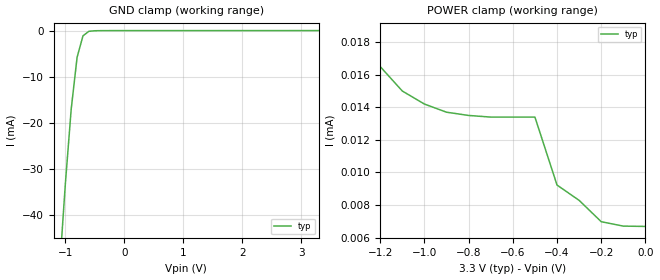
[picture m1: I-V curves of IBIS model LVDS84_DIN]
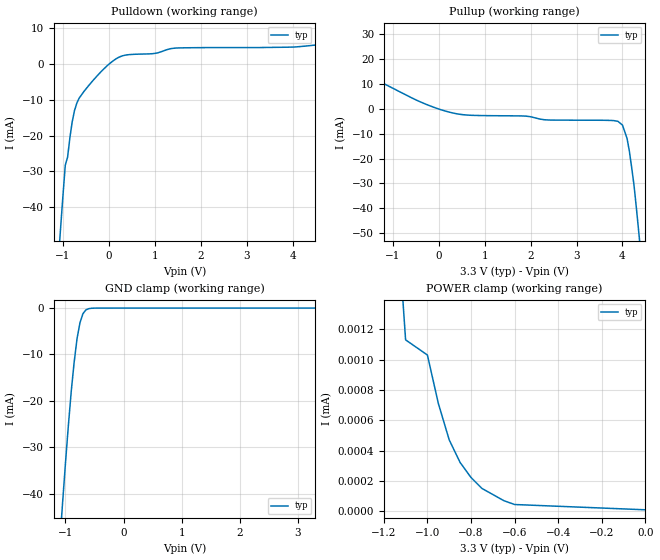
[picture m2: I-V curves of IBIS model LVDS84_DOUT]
|   Texas Instruments Incorporated
|   Data Transmissions Products
|   IBIS Model for SN75LVDS84
|   48DGG Package
[IBIS Ver]   2.1
[Comment char]   |_char
[File name]   75lvds84.ibs
[File Rev]   2.0
[Date]   21Feb97
[Source]   File originated at Texas Instruments Incorporated.
   Data Transmission Products Group. All data based on
   Empirical Measurements(Bench).
[Notes]   File created by Thomas Fisher
[Disclaimer]
(C) Copyright Texas Instruments Incorporated 1997
   All rights reserved
  Texas Instruments Incorporated hereby grants the user of this IBIS
model a non-exclusive, nontransferable license to use this IBIS model
under the following terms.  Before using this IBIS model, the user
should read this license.  If the user does not accept these terms,
the IBIS model should be returned to Texas Instruments within 30 days.
  The user is granted this license only to use the IBIS model and
is not granted rights to sell, load, rent, lease or license the IBIS
model in whole or in part, or in modified form to anyone other than
user.  User may modify the IBIS model to suit its specific applications
but rights to derivative works and such modifications shall belong to
Texas Instruments.
  This IBIS model is provided on an "AS IS" basis and Texas Instruments
makes absolutely no warranty with respect to the information contained
herein.  TEXAS INSTRUMENTS DISCLAIMS AND CUSTOMER WAIVES ALL WARRANTIES,
EXPRESS OR IMPLIED, INCLUDING WARRANTIES OF MERCHANTABILITY OR FITNESS
FOR A PARTICULAR PURPOSE. The entire risk as to quality and performance
is with the Customer. ACCORDINGLY, IN NO EVENT SHALL THE COMPANY BE LIABLE
FOR ANY DAMAGES, WHETHER IN CONTRACT OR TORT,INCLUDING ANY LOST PROFITS
OR OTHER INCIDENTAL, CONSEQUENTIAL, EXEMPLARY, OR PUNITIVE DAMAGES ARISING
OUT OF THE USE OR APPLICATION OF THE IBIS model provided in this package.
Further, Texas Instruments reserves the right to discontinue or make changes
without notice to any product herein to improve reliability, function, or
design. Texas Instruments does not convey any license under patent rights
or any other intellectual property rights, including those of third parties.
Contact Texas Instruments at ATTN:DATA TRANSMISSIONS
Thomas Fisher  8505 Forest Lane, M/S 8710, Dallas, TX 75243-4136
IBIS Open Forum disclaims all warranties. See DISCLAIM.TXT
in vhdl.org:/pub/IBIS/models for the full disclaimer.
[Copyright]   Copyright 1997, Texas Instruments, All Rights Reserved
[Component]   SN75LVDS84DGG
[Manufacturer]  Texas Instruments Incorporated
[Package]
|   typ   min   max
R_pkg   0.036   0.022   0.041
L_pkg   2.128nH   2.045nH   2.336nH
C_pkg   0.357pF   0.310pF   0.394pF
[Pin]  signal_name   model_name   R_pin   L_pin   C_pin
1   D4   LVDS84_DIN   0.041   2.221n   0.310p
2   VCC   POWER   0.041   2.297n   0.394p
3   D5   LVDS84_DIN   0.022   2.336n   0.380p
4   D6   LVDS84_DIN   0.031   2.056n   0.343p
5   GND   GND   0.034   2.099n   0.383p
6   D7   LVDS84_DIN   0.034   2.046n   0.360p
7   D8   LVDS84_DIN   0.036   2.052n   0.354p
8   VCC   POWER   0.038   2.081n   0.354p
9   D9   LVDS84_DIN   0.039   2.091n   0.353p
10   D10   LVDS84_DIN   0.039   2.068n   0.349p
11   GND   GND   0.039   2.098n   0.361p
12   D11   LVDS84_DIN   0.039   2.100n   0.343p
13   D12   LVDS84_DIN   0.039   2.100n   0.343p
14   VCC   POWER   0.039   2.098n   0.361p
15   D13   LVDS84_DIN   0.039   2.068n   0.349p
16   D14   LVDS84_DIN   0.039   2.091n   0.353p
17   GND   GND   0.038   2.081n   0.354p
18   D15   LVDS84_DIN   0.036   2.052n   0.354p
19   D16   LVDS84_DIN   0.034   2.045n   0.360p
20   D17   LVDS84_DIN   0.034   2.099n   0.383p
21   VCC   POWER   0.031   2.056n   0.343p
22   D18   LVDS84_DIN   0.022   2.330n   0.381p
23   D19   LVDS84_DIN   0.041   2.294n   0.394p
24   GND   GND   0.041   2.220n   0.310p
25   D20   LVDS84_DIN   0.041   2.221n   0.310p
26   CLKIN   LVDS84_DIN   0.041   2.295n   0.394p
27   SHTDN   LVDS84_DIN   0.022   2.333n   0.378p
28   PLLGND   GND   0.031   2.056n   0.343p
29   PLLVCC   POWER   0.034   2.097n   0.385p
30   PLLGND   GND   0.034   2.045n   0.360p
31   LVDSGND   GND   0.036   2.052n   0.354p
32   CLKOUTP   LVDS84_DOUT   0.038   2.080n   0.354p
33   CLKOUTM   LVDS84_DOUT   0.039   2.090n   0.352p
34   Y2P   LVDS84_DOUT   0.039   2.067n   0.349p
35   Y2M   LVDS84_DOUT   0.039   2.097n   0.362p
36   LVDSGND   GND   0.039   2.100n   0.343p
37   LVDSVCC   POWER   0.039   2.100n   0.343p
38   Y1P   LVDS84_DOUT   0.039   2.097n   0.362p
39   Y1M   LVDS84_DOUT   0.039   2.067n   0.349p
40   Y0P   LVDS84_DOUT   0.039   2.090n   0.352p
41   Y0M   LVDS84_DOUT   0.038   2.080n   0.354p
42   LVDSGND   GND   0.036   2.052n   0.354p
43   NC   NC
44   D0   LVDS84_DIN   0.034   2.097n   0.385p
45   D1   LVDS84_DIN   0.031   2.056n   0.343p
46   GND   GND   0.022   2.335n   0.377p
47   D2   LVDS84_DIN   0.041   2.297n   0.394p
48   D3   LVDS84_DIN   0.041   2.221n   0.310p
[Diff_pin]   inv_pin   vdiff   tdelay_typ   tdelay_min   tdelay_max
| The 'YXP' pin is Diff_pin and the 'YXM' pin is the inv_pin
| The 'CLKOUTP' pin is Diff_pin and the 'CLKOUTM' pin is the inv_pin
32   33   NA   0 0 0
34   35   NA   0 0 0
38   39   NA   0 0 0
40   41   NA   0 0 0
| Models and submodels in the file (2): LVDS84_DIN (Input), LVDS84_DOUT (3-state)
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|   Driver Input  MODEL
[Model]   LVDS84_DIN
Model_type   Input
|Signals   D0,D1,D2,D3,D4,D5,D6,D7,D8,D9,D10,D11,D12,D13,D14,D15,D16,
|   D17,D18,D19,D20,SHTDN,CLKIN
Vinh = 2.0
Vinl = 0.8
|   typ   min   max
C_comp   1.0pF   NA   NA
|   typ   min   max
[Temperature Range]   25.0   NA   NA
[Voltage range]   3.3V   3.0V   3.6V
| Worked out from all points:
|   GND clamp passes 1 mA (typ) near -0.69 V on its own axis
[Power_clamp]
| Note that the[POWER_clamp]voltage table is referenced to Vcc
| and is calculated using Vtable=Vcc - Vmeasured.
|   Voltage   I(typ)   I(min)   I(max)
-3.3V     780uA      NA         NA
-1.3V     19.1uA     NA         NA
-1.2V     16.5uA     NA         NA
-1.1V     15uA       NA         NA
-1V       14.2uA     NA         NA
-900mV    13.7uA     NA         NA
-800mV    13.5uA     NA         NA
-500mV    13.4uA     NA         NA
-400mV    9.23uA     NA         NA
-300mV    8.29uA     NA         NA
-200mV    6.98uA     NA         NA
0V        6.69uA     NA         NA
[GND_clamp]
|   Voltage   I(typ)   I(min)   I(max)
-3.3V     -485.8mA   NA         NA
-1.1V     -52.3mA    NA         NA
-1V       -33.38mA   NA         NA
-900mV    -17.03mA   NA         NA
-800mV    -5.78mA    NA         NA
-700mV    -1.13mA    NA         NA
-600mV    -150uA     NA         NA
-300mV    -2.96uA    NA         NA
3.3V      6.69uA     NA         NA
|   Driver Output  MODEL
[Model]   LVDS84_DOUT
Model_type   3-state
| Signals   Y0P,Y0M,Y1P,Y1M,Y2P,Y2M,CLKOUTP,CLKOUTM
Vmeas = 1.2V   |Reference voltage for timing measurements
Cref = 5pF   |Timing specification test load capacitance value
Rref = 50   |Note: 50 Ohm load; single ended configuration
Vref = 1.18V   |Timing specification test load voltage
| variable   typ   min   max
C_comp   1.0pF   NA   NA
|   typ   min   max
[Temperature Range]   25.0   NA   NA
[Voltage range]   3.3V   3.0V   3.6V
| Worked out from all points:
|   slope of the pulldown table from 0 to 0.495 V, typ, clamps not added: 182 ohm
|   slope of the pullup table from 0 to 0.495 V, typ, clamps not added: 224 ohm
|   GND clamp passes 1 mA (typ) near -0.69 V on its own axis
[Pulldown]
|   Voltage   I(typ)   I(min)   I(max)
-3.3V     -466.3mA   NA         NA
-1.1V     -54.41mA   NA         NA
-1.05V    -45.42mA   NA         NA
-950mV    -28.23mA   NA         NA
-900mV    -26.02mA   NA         NA
-800mV    -16.18mA   NA         NA
-700mV    -10.96mA   NA         NA
-250mV    -3.21mA    NA         NA
250mV     2.077mA    NA         NA
1.45V     4.458mA    NA         NA
4.15V     4.857mA    NA         NA
6.6V      9.522mA    NA         NA
[Pullup]
|   Voltage   I(typ)   I(min)   I(max)
| Note that the[Pullup]voltage table is referenced to Vcc
| and is calculated using Vtable=Vcc - Vmeasured.
-3.3V     32.52mA    NA         NA
-1.3V     11.15mA    NA         NA
200mV     -1.15mA    NA         NA
2.4V      -4.46mA    NA         NA
3.9V      -4.96mA    NA         NA
4V        -6.51mA    NA         NA
4.1V      -11.9mA    NA         NA
4.15V     -17.01mA   NA         NA
4.25V     -30.57mA   NA         NA
4.35V     -48.72mA   NA         NA
4.4V      -58.4mA    NA         NA
6.6V      -501.5mA   NA         NA
[GND_clamp]
|   Voltage   I(typ)   I(min)   I(max)
| Outputs in Tri-state.
-3.3V     -462.7mA   NA         NA
-1.1V     -51.07mA   NA         NA
-1.05V    -42.1mA    NA         NA
-950mV    -25.35mA   NA         NA
-900mV    -17.89mA   NA         NA
-850mV    -11.64mA   NA         NA
-800mV    -6.53mA    NA         NA
-750mV    -3.14mA    NA         NA
-700mV    -1.23mA    NA         NA
-650mV    -410uA     NA         NA
-450mV    -2.68uA    NA         NA
3.3V      16.9nA     NA         NA
[POWER_clamp]
|   Voltage   I(typ)   I(min)   I(max)
| Note that the [POWER_clamp] voltage table is referenced to Vcc
| and is calculated using Vtable = Vcc - Vmeasured.
| Outputs in Tri-state.
-3.3V     729uA      NA         NA
-1.15V    2.18uA     NA         NA
-1.1V     1.13uA     NA         NA
-1V       1.03uA     NA         NA
-950mV    712nA      NA         NA
-900mV    471nA      NA         NA
-850mV    322nA      NA         NA
-800mV    223nA      NA         NA
-750mV    151nA      NA         NA
-650mV    70.7nA     NA         NA
-600mV    45nA       NA         NA
0V        10.2nA     NA         NA
[Ramp]
| Note: Ramp rate measured on single-ended Driver Output.
|   typ   min   max
dV/dt_r   0.200/258ps   NA   NA
dV/dt_f   0.200/250ps   NA   NA
R_load = 100ohm | Note: These are single ended driver measurements
